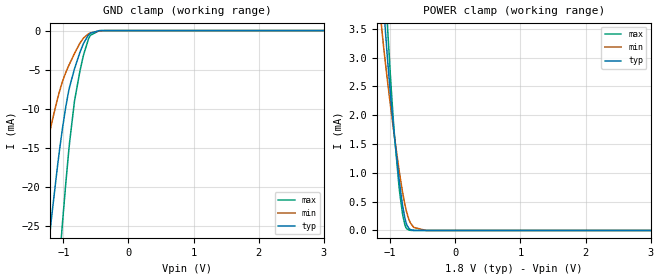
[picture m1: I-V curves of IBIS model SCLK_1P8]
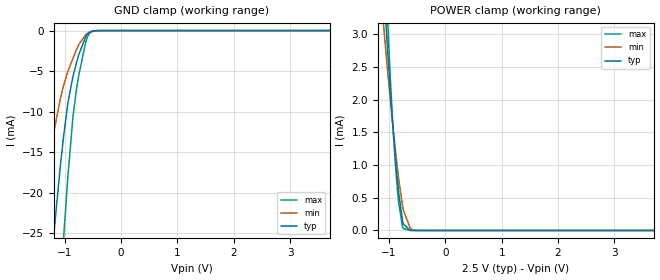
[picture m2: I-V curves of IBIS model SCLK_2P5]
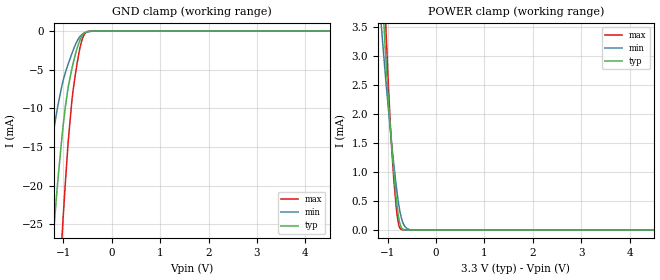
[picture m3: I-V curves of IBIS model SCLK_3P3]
| Texas Instruments Incorporated
| High-Resolution Analog to Digital Converter
| Marketing part#   Voltage Range   Package-type   #pins/pkg drawing
| ADS1262IPW   1.65V - 3.6V   TSSOP   28-pin PW
[IBIS Ver]   4.1
[File name]   ads1262.ibs
[File Rev]   1.0
[Date]   01/26/2015
[Source]   Model built from spectre simulations at:
   Texas Instruments Incorporated.
   Analog-eLab, HPA
   12500 TI Blvd
   Dallas, TX -75243
   For Support e-mail: elab_ibis@list.ti.com
[Notes]   Revision History
   Rev 1.0: 01/26/2015
   - ccomp values are based on PVT settings:
   MIN: Low Voltage, High Temperature, Weak Process
   TYP: Nominal Voltage, Nominal Temperature, Nominal Process
   MAX: High Voltage, Low Temperature, Fast Process
   - C_comp although listed in numerical order of value are obtained from varying PVT conditions.
   For PVT conditions for each specific value, refer to the buffer description under respective [Model].
   IBIS model user is responsible for using appropriate C_comp to simulate for Signal Integrity.
[Disclaimer]  This model is designed as an aid for customers of Texas Instruments
 TI and its licensors and suppliers make no warranties, either expressed
 or implied, with respect to this  model, including the warranties of
 merchantability or fitness for a particular purpose.
 The model is provided solely on an "as is" basis. The entire risk as to
 its quality and performance is with the customer.
[Copyright] (C)Copyright 2015 Texas Instruments Incorporated.
   All rights reserved.
[Component]   ADS1262IPW
[Manufacturer]  Texas Instruments Incorporated
[Package]   |28-pin PW TSSOP package
|   typ   min   max
R_pkg   0.1269   0.0756   0.1873
L_pkg   1.3818n   0.8765n   2.1775n
C_pkg   0.4353p   0.3806p   0.5160p
[Pin]   signal_name   model_name   R_pin   L_pin   C_pin
1   AIN8   NC   0.18725  2.17751n  0.51382p
2   AIN9   NC   0.15344  1.71317n  0.47897p
3   AINCOM   NC   0.11801  1.23544n  0.40827p
4   CAPP   NC   0.11461  1.17103n  0.41165p
5   CAPN   NC   0.11546  1.18455n  0.41511p
6   AVDD   POWER   0.08587  0.96561n  0.42376p
7   AVSS   GND   0.07613  0.88756n  0.42626p
8   REFOUT   NC   0.07558  0.87652n  0.43340p
9   START   RESET   0.11026  1.11783n  0.38057p
10   CSB   RESET   0.10972  1.11740n  0.41054p
11   SCLK   SCLK   0.11105  1.13449n  0.40609p
12   DIN   RESET   0.11638  1.20941n  0.40724p
13   DOUT   DOUT   0.14921  1.72076n  0.47881p
14   DRDY   DRDY   0.17909  2.09903n  0.51450p
15   CLIN   SCLK   0.17989  2.13481n  0.51596p
16   XTAL2   NC   0.16062  1.73050n  0.48364p
17   BYPASS   NC   0.12014  1.28639n  0.41219p
18   DGND   GND   0.10891  1.13617n  0.41168p
19   DVDD   POWER   0.10833  1.12227n  0.41107p
20   RESETB   RESET   0.10868  1.12885n  0.39369p
21   AIN0   NC   0.13726  1.53739n  0.41611p
22   AIN1   NC   0.11911  1.25386n  0.40285p
23   AIN2   NC   0.12513  1.33839n  0.40359p
24   AIN3   NC   0.11556  1.18080n  0.41499p
25   AIN4   NC   0.11119  1.11560n  0.40894p
26   AIN5   NC   0.11955  1.26330n  0.41125p
27   AIN6   NC   0.14973  1.67674n  0.47865p
28   AIN7   NC   0.18665  2.17508n  0.51391p
[Model Selector] SCLK
SCLK_3P3   SCLK Input buffer, 3.3V supply
SCLK_2P5   SCLK Input buffer, 2.5V supply
SCLK_1P8   SCLK Input buffer, 1.8V supply
[Model Selector] RESET
RESET_3P3   RESET Input buffer, 3.3V supply
RESET_2P5   RESET Input buffer, 2.5V supply
RESET_1P8   RESET Input buffer, 1.8V supply
[Model Selector] DOUT
DOUT_3P3   DOUT Input buffer, 3.3V supply
DOUT_2P5   DOUT Input buffer, 2.5V supply
DOUT_1P8   DOUT Input buffer, 1.8V supply
[Model Selector] DRDY
DRDY_3P3   DRDY Input buffer, 3.3V supply
DRDY_2P5   DRDY Input buffer, 2.5V supply
DRDY_1P8   DRDY Input buffer, 1.8V supply
| Models and submodels in the file (12): SCLK_1P8 (Input), SCLK_2P5 (Input), SCLK_3P3 (Input), RESET_1P8 (Input), RESET_2P5 (Input), RESET_3P3 (Input), DOUT_3P3 (3-state), DOUT_2P5 (3-state), DOUT_1P8 (3-state), DRDY_3P3 (Output), DRDY_2P5 (Output), DRDY_1P8 (Output)
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|   Model SCLK_1P8
[Model]   SCLK_1P8
Model_type   Input
Vinl = 0.36
Vinh = 1.44
|   typ   min   max
|   (nom PVT)   (fast PVT)   (slow PVT)
C_comp   0.205pF   0.203pF   0.216pF
[Model spec]
|subparameter
Vinl   0.36   0.33   0.39
Vinh   1.44   1.32   1.56
[Voltage Range]   1.8   1.65   1.95
[Temperature Range]   27   125   -40
[Power Clamp Reference]   1.8   1.65   1.95
[GND Clamp Reference]   -0   -0   -0
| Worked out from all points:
|   GND clamp passes 1 mA (typ) near -0.64 V on its own axis
|   POWER clamp passes 1 mA (typ) near -0.87 V on its own axis
[GND Clamp]
|   Voltage   I(typ)   I(min)   I(max)
-1.8V     -80.71mA   -43.38mA   -120.5mA
-1.557V   -56.83mA   -29.44mA   -89.71mA
-1.417V   -43.81mA   -22.24mA   -72.1mA
-1.217V   -26.83mA   -13.36mA   -47.69mA
-1.174V   -23.49mA   -11.69mA   -42.59mA
-1.022V   -13.12mA   -6.787mA   -25.7mA
-914.4mV  -7.645mA   -4.457mA   -15.27mA
-828mV    -4.902mA   -2.941mA   -9.04mA
-693mV    -1.711mA   -994.9uA   -3.251mA
-612mV    -549.1uA   -410.3uA   -1.04mA
-433.8mV  -7.963uA   -38.8uA    -7.561uA
3.595V    0A         0A         0A
[POWER Clamp]
|   Voltage   I(typ)   I(min)   I(max)
-1.8V     16.9mA     12.99mA    20.87mA
-1.174V   5.114mA    3.995mA    6.361mA
-1.093V   3.763mA    3.105mA    4.608mA
-1.049V   3.103mA    2.675mA    3.714mA
-1.039V   2.946mA    2.571mA    3.498mA
-946.8mV  1.771mA    1.735mA    1.842mA
-865.8mV  916.1uA    1.068mA    783.8uA
-806.4mV  412.7uA    643.7uA    263.5uA
-741.6mV  89.99uA    295.6uA    25.79uA
-639mV    2.274uA    54.53uA    163.5nA
-450mV    0A         407nA      0A
3.595V    0A         0A         0A
|   Model SCLK_2P5
[Model]   SCLK_2P5
Model_type   Input
Vinl = 0.50
Vinh = 2.00
|   typ   min   max
|   (nom PVT)   (fast PVT)   (slow PVT)
C_comp   0.211pF   0.208pF   0.222pF
[Model spec]
|subparameter
Vinl   0.50   0.45   0.55
Vinh   2.00   1.80   2.20
[Voltage Range]   2.5   2.25   2.75
[Temperature Range]   27   125   -40
[Power Clamp Reference]   2.5   2.25   2.75
[GND Clamp Reference]   -0   -0   -0
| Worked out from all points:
|   GND clamp passes 1 mA (typ) near -0.64 V on its own axis
|   POWER clamp passes 1 mA (typ) near -0.87 V on its own axis
[GND Clamp]
|   Voltage   I(typ)   I(min)   I(max)
-2.5V     -154mA     -90.46mA   -209.7mA
-1.472V   -48.91mA   -25.02mA   -79.08mA
-1.195V   -25.13mA   -12.51mA   -45.11mA
-1.083V   -16.95mA   -8.54mA    -32.2mA
-1.022V   -13.12mA   -6.791mA   -25.71mA
-940mV    -8.729mA   -4.935mA   -17.55mA
-857.5mV  -5.747mA   -3.451mA   -10.84mA
-797.5mV  -4.086mA   -2.427mA   -7.5mA
-752.5mV  -2.974mA   -1.725mA   -5.519mA
-625mV    -684uA     -477.3uA   -1.306mA
-542.5mV  -133.1uA   -177.9uA   -218.6uA
4.992V    0A         0A         0A
[POWER Clamp]
|   Voltage   I(typ)   I(min)   I(max)
-2.5V     30.6mA     23.86mA    37.48mA
-1.097V   3.842mA    3.156mA    4.712mA
-1.045V   3.039mA    2.633mA    3.626mA
-1.03V    2.825mA    2.49mA     3.328mA
-977.5mV  2.136mA    2.007mA    2.35mA
-925mV    1.527mA    1.549mA    1.517mA
-865mV    909uA      1.062mA    775.3uA
-827.5mV  574.9uA    786.3uA    421.2uA
-745mV    99.61uA    310.7uA    30.02uA
-625mV    1.316uA    41.69uA    66.23nA
-505mV    0A         2.059uA    0A
4.992V    0A         0A         0A
|   Model SCLK_3P3
[Model]   SCLK_3P3
Model_type   Input
Vinl = 0.66
Vinh = 2.64
|   typ   min   max
|   (nom PVT)   (fast PVT)   (slow PVT)
C_comp   0.213pF   0.211pF   0.214pF
[Model spec]
|subparameter
Vinl   0.66   0.60   0.72
Vinh   2.64   2.40   2.88
[Voltage Range]   3.3   3   3.6
[Temperature Range]   27   125   -40
[Power Clamp Reference]   3.3   3   3.6
[GND Clamp Reference]   -0   -0   -0
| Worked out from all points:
|   GND clamp passes 1 mA (typ) near -0.65 V on its own axis
|   POWER clamp passes 1 mA (typ) near -0.87 V on its own axis
[GND Clamp]
|   Voltage   I(typ)   I(min)   I(max)
-3.3V     -240.4mA   -150.9mA   -311mA
-1.488V   -50.37mA   -25.83mA   -81.06mA
-1.231V   -27.95mA   -13.93mA   -49.38mA
-1.142V   -21.12mA   -10.53mA   -38.9mA
-1.033V   -13.76mA   -7.073mA   -26.81mA
-1.013V   -12.57mA   -6.547mA   -24.74mA
-904.2mV  -7.262mA   -4.274mA   -14.41mA
-825mV    -4.821mA   -2.892mA   -8.879mA
-666.6mV  -1.252mA   -757.8uA   -2.397mA
-607.2mV  -504.5uA   -388.8uA   -951.9uA
-537.9mV  -119.6uA   -168uA     -193.4uA
6.59V     0A         0A         0A
[POWER Clamp]
|   Voltage   I(typ)   I(min)   I(max)
-3.3V     46.32mA    36.4mA     56.46mA
-1.132V   4.405mA    3.523mA    5.45mA
-1.102V   3.918mA    3.205mA    4.812mA
-1.053V   3.152mA    2.708mA    3.782mA
-1.043V   3.008mA    2.613mA    3.583mA
-943.8mV  1.737mA    1.711mA    1.796mA
-874.5mV  1.001mA    1.137mA    878.3uA
-795.3mV  337.5uA    575.5uA    195.4uA
-716.1mV  39.41uA    204.1uA    7.813uA
-627mV    1.414uA    43.54uA    67.93nA
-478.5mV  0A         939.2nA    0A
6.59V     0A         0A         0A
